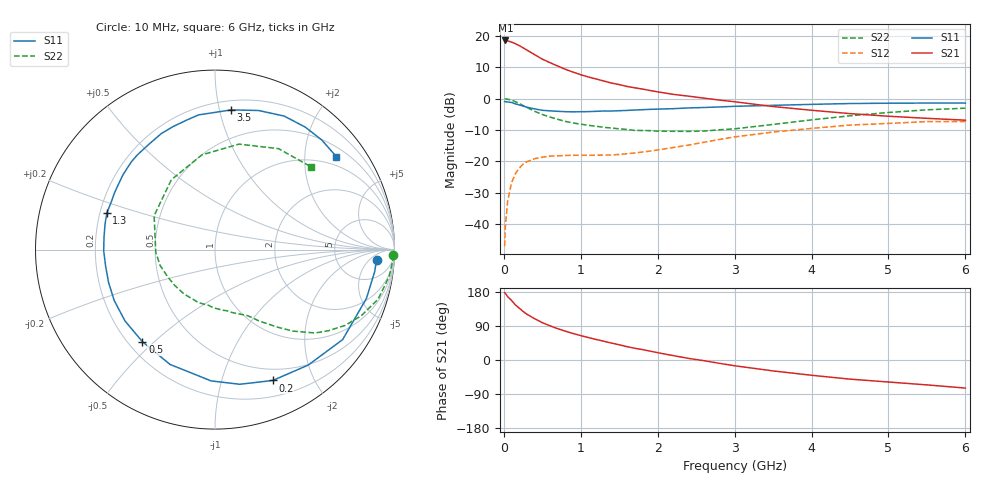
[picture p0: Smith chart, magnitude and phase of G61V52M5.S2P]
! SIEMENS Small Signal Semiconductors
! BFG193
! Si NPN RF Bipolar Junction Transistor in SOT223
! VCE = 1.5 V  IC = 2.5 mA
! Common Emitter S-Parameters:  August  1996
# GHz  S  MA  R  50
!  f  S11  S21  S12  S22
! GHz  MAG  ANG  MAG  ANG  MAG  ANG  MAG  ANG
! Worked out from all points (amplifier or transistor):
!   36 points, 10 MHz to 6 GHz, reference 50 ohm
!   highest |S21| = 18.6 dB at 20 MHz (marker M1)
!   |S21| within 3 dB of that: start of sweep to 294.8 MHz
!   unconditionally stable (mu >= 1): 1.314 GHz to 2.802 GHz
!   at 250 MHz: K = 0.21, MSG = 18.6 dB, |S12| = -20.9 dB
!   at 1.4 GHz: K = 1.07, MAG = 9.9 dB, |S12| = -18.0 dB
!   at 6 GHz: K = 0.98, MSG = 0.2 dB, |S12| = -7.3 dB
!   S11 on the Smith chart (normalised r, x): 10 MHz: 14, -9; 200 MHz: 0.37, -1.47; 500 MHz: 0.26, -0.46; 1.3 GHz: 0.23, +0.16; 3.5 GHz: 0.27, +1.09; 6 GHz: 0.73, +2.77
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0.01  0.9018 -3.6  8.446 177.5  0.0044 92.4  0.9935 -1.8
0.02  0.8984 -7.7  8.533 175.9  0.0092 85.5  0.9924 -3.5
0.05  0.8865 -17.9  8.393 167.2  0.0233 79.8  0.9816 -8.8
0.1  0.8701 -35.2  8.053 157.3  0.0453 71.4  0.95 -16.9
0.15  0.8268 -51.1  7.563 145.4  0.0632 61.9  0.8945 -24.3
0.2  0.797 -66.2  7.058 136.9  0.0777 55.3  0.8393 -30.2
0.25  0.7628 -79.6  6.512 128.1  0.0898 48.7  0.7767 -35.6
0.3  0.7319 -91.7  5.989 120.7  0.0984 43.7  0.7258 -39.8
0.4  0.6871 -111.4  5.062 109.1  0.1099 35.7  0.6292 -46.2
0.5  0.6533 -128.2  4.294 98.5  0.1164 29.6  0.5596 -50.8
0.6  0.6399 -141.6  3.768 90.2  0.1211 25.8  0.5089 -54.5
0.7  0.6291 -153.2  3.331 82.7  0.1222 22.9  0.4685 -58.2
0.9  0.6164 -171.5  2.661 69.9  0.1249 19.5  0.4097 -63.9
1.1  0.6221 173.8  2.223 59.2  0.1248 18.4  0.3759 -71.3
1.3  0.6363 161.2  1.915 49.4  0.126 19.1  0.3485 -78.4
1.7  0.66 141.2  1.497 31.1  0.1358 23.0  0.3117 -96.9
2.2  0.693 122.0  1.175 11.7  0.1658 24.7  0.3016 -124.8
2.8  0.7387 102.3  0.952 -8.7  0.2231 20.5  0.3184 -164.0
3.5  0.7835 83.4  0.75 -28.8  0.2933 6.3  0.3881 150.9
4.5  0.8378 62.6  0.578 -50.5  0.3789 -15.4  0.533 97.8
5.5  0.8525 45.8  0.486 -65.7  0.4306 -41.5  0.6646 57.8
6  0.8517 37.5  0.454 -74.1  0.4318 -55.9  0.7062 40.8
